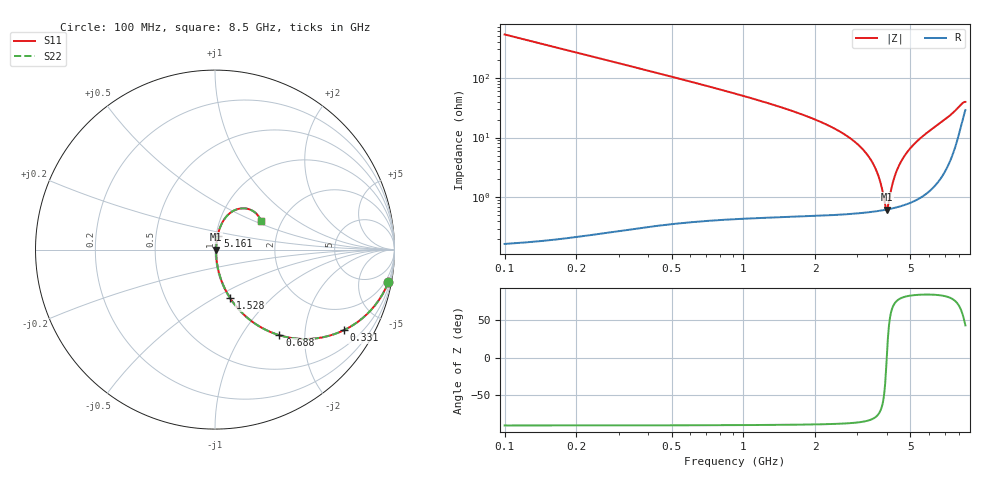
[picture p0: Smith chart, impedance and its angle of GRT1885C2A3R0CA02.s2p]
!Murata Part Number: GRT1885C2A3R0CA02
!These Parameters are Measured in Series Mode Connection
!Data Generated on Jun 19, 2026
!  o--ll--o
!Port1  Port2
!  o------o
!Operation Temp=25[degC], DC Bias Voltage=0[V]
!Freq. Start=100[MHz] Stop=9[GHz] 401[Steps]
# Hz S RI R 50
!Freq.(Hz) S11(Real) S11(Imag) S21(Real) S21(Imag) S12(Real) S12(Imag) S22(Real) S22(Imag)
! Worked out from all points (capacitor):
!   401 points, 100 MHz to 8.5 GHz, reference 50 ohm
!   read as one part in series: C = 3 pF near 142 MHz
!   lowest |Z| = 627 mohm at 3.985 GHz (marker M1)
!   series resonance near 3.981 GHz, so ESL is about 530 pH
!   S11 on the Smith chart (normalised r, x): 100 MHz: 1, -11; 331 MHz: 1.01, -3.18; 688 MHz: 1.01, -1.50; 1.528 GHz: 1.01, -0.59; 5.161 GHz: 1.02, +0.15; 8.5 GHz: 1.58, +0.54
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1e8  0.9656 -0.1821  0.0344 0.1821  0.0344 0.1821  0.9656 -0.1821
2.26e8  0.8452 -0.3612  0.1548 0.3612  0.1548 0.3612  0.8452 -0.3612
3.31e8  0.7163 -0.4499  0.2837 0.4499  0.2837 0.4499  0.7163 -0.4499
4.78e8  0.5441 -0.4965  0.4559 0.4965  0.4559 0.4965  0.5441 -0.4965
6.88e8  0.3592 -0.4771  0.6408 0.4771  0.6408 0.4771  0.3592 -0.4771
1.024e9  0.192 -0.3893  0.808 0.3893  0.808 0.3893  0.192 -0.3893
1.507e9  0.0874 -0.2747  0.9126 0.2747  0.9126 0.2747  0.0874 -0.2747
1.528e9  0.0846 -0.2705  0.9154 0.2705  0.9154 0.2705  0.0846 -0.2705
2.914e9  0.0126 -0.0845  0.9874 0.0845  0.9874 0.0845  0.0126 -0.0845
3.292e9  0.00825 -0.0515  0.9918 0.0515  0.9918 0.0515  0.00825 -0.0515
3.565e9  0.0067 -0.03  0.9933 0.03  0.9933 0.03  0.0067 -0.03
3.733e9  0.00626 -0.0176  0.9937 0.0176  0.9937 0.0176  0.00626 -0.0176
3.922e9  0.00617 -0.00411  0.9938 0.00411  0.9938 0.00411  0.00617 -0.00411
3.985e9  0.00623 0.000245  0.9938 -0.000245  0.9938 -0.000245  0.00623 0.000245
4.027e9  0.00629 0.00312  0.9937 -0.00312  0.9937 -0.00312  0.00629 0.00312
4.3e9  0.0071 0.0213  0.9929 -0.0213  0.9929 -0.0213  0.0071 0.0213
4.636e9  0.00905 0.0425  0.991 -0.0425  0.991 -0.0425  0.00905 0.0425
5.161e9  0.0141 0.0741  0.9859 -0.0741  0.9859 -0.0741  0.0141 0.0741
5.707e9  0.0222 0.106  0.9778 -0.106  0.9778 -0.106  0.0222 0.106
7.114e9  0.0692 0.1906  0.9308 -0.1906  0.9308 -0.1906  0.0692 0.1906
8.017e9  0.1711 0.2291  0.8289 -0.2291  0.8289 -0.2291  0.1711 0.2291
8.5e9  0.2566 0.1566  0.7434 -0.1566  0.7434 -0.1566  0.2566 0.1566
